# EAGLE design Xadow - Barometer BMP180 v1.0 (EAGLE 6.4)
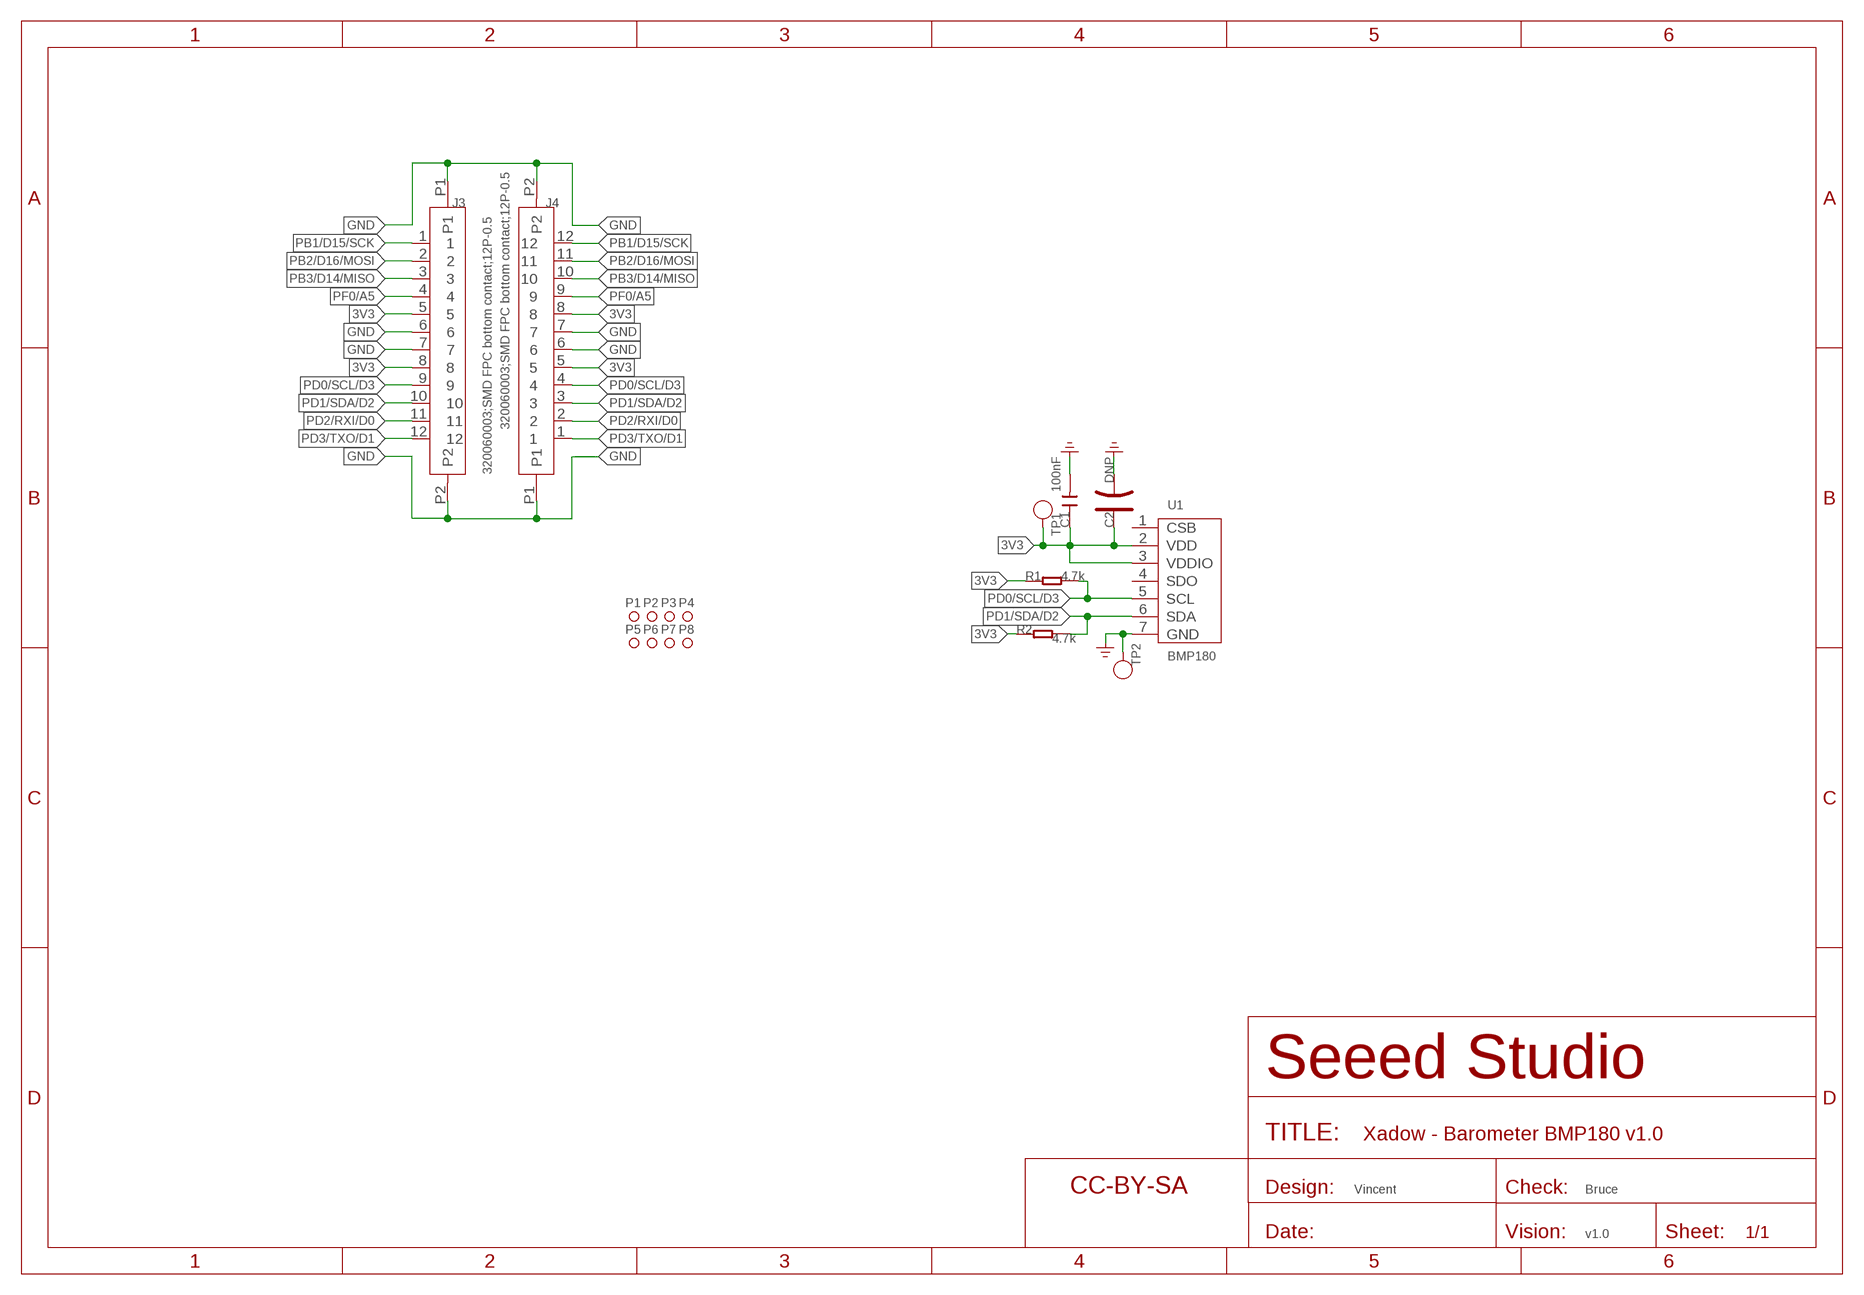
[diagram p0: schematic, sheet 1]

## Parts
C1  100nF  CAP-0603  [C0603]
C2  DNP  CAP-POLAR-AVX-A  [AVX-A]
J3  320060003;SMD FPC bottom contact;12P-0.5  FPC-CONNECTOR-12P-FH12-12S-0.5SH  [12P-0.5]
J4  320060003;SMD FPC bottom contact;12P-0.5  FPC-CONNECTOR-12P-FH12-12S-0.5SH  [12P-0.5]
P1  PAD-MARK'ANNULAR'  [ROUND-MARK-1.0]
P2  PAD-MARK'ANNULAR'  [ROUND-MARK-1.0]
P3  PAD-MARK'ANNULAR'  [ROUND-MARK-1.0]
P4  PAD-MARK'ANNULAR'  [ROUND-MARK-1.0]
P5  PAD-MARK'ANNULAR'  [ROUND-MARK-1.0]
P6  PAD-MARK'ANNULAR'  [ROUND-MARK-1.0]
P7  PAD-MARK'ANNULAR'  [ROUND-MARK-1.0]
P8  PAD-MARK'ANNULAR'  [ROUND-MARK-1.0]
R1  4.7k  RES-0603  [R0603]
R2  4.7k  RES-0603  [R0603]
TP1  PAD-TEST-POINT'4545'  [TP-D45MIL]
TP2  PAD-TEST-POINT'4545'  [TP-D45MIL]
U1  BMP180  [LGA-7]
U$1  SEEEDSTUDIO-OPEN-SCH-FRAME  [SEEEDSTUDIO-PCB-FRAME]

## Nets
3V3: C1.1 C2.+ J3.5 J3.8 J4.5 J4.8 R1.1 R2.1 TP1.T U1.2(VDD) U1.3(VDDIO)
GND: C1.2 C2.- J3.6 J3.7 J3.P1 J3.P2 J4.6 J4.7 J4.P1 J4.P2 TP2.T U1.7(GND) ; supply symbol labelled GND_POWER
PB1/D15/SCK: J3.1 J4.12
PB2/D16/MOSI: J3.2 J4.11
PB3/D14/MISO: J3.3 J4.10
PD0/SCL/D3: J3.9 J4.4 R1.2 U1.5(SCL)
PD1/SDA/D2: J3.10 J4.3 R2.2 U1.6(SDA)
PD2/RXI/D0: J3.11 J4.2
PD3/TXO/D1: J3.12 J4.1
PF0/A5: J3.4 J4.9
Unconnected: U1.1(CSB) U1.4(SDO)

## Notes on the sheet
- Vincent | Bruce
- v1.0

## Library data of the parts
C1 = Discrete-new:CAP: Ceramic Capacitors
C2 = Discrete-new:CAP-POLAR: Electrolytic Capacitors,Tantalum Capacitors and Super Capacitors
J3 J4 = Connector-new:FPC-CONNECTOR-12P: 320060003
P1-P8 = Discrete-new:PAD-MARK; PARTNO: DNP
R1 R2 = Discrete-new:RES
TP1 TP2 = Discrete-new:PAD-TEST-POINT; PARTNO: DNP
U1 = template:BMP180: Digital pressure sensor
U$1 = moudle-new:SEEEDSTUDIO-OPEN-SCH-FRAME

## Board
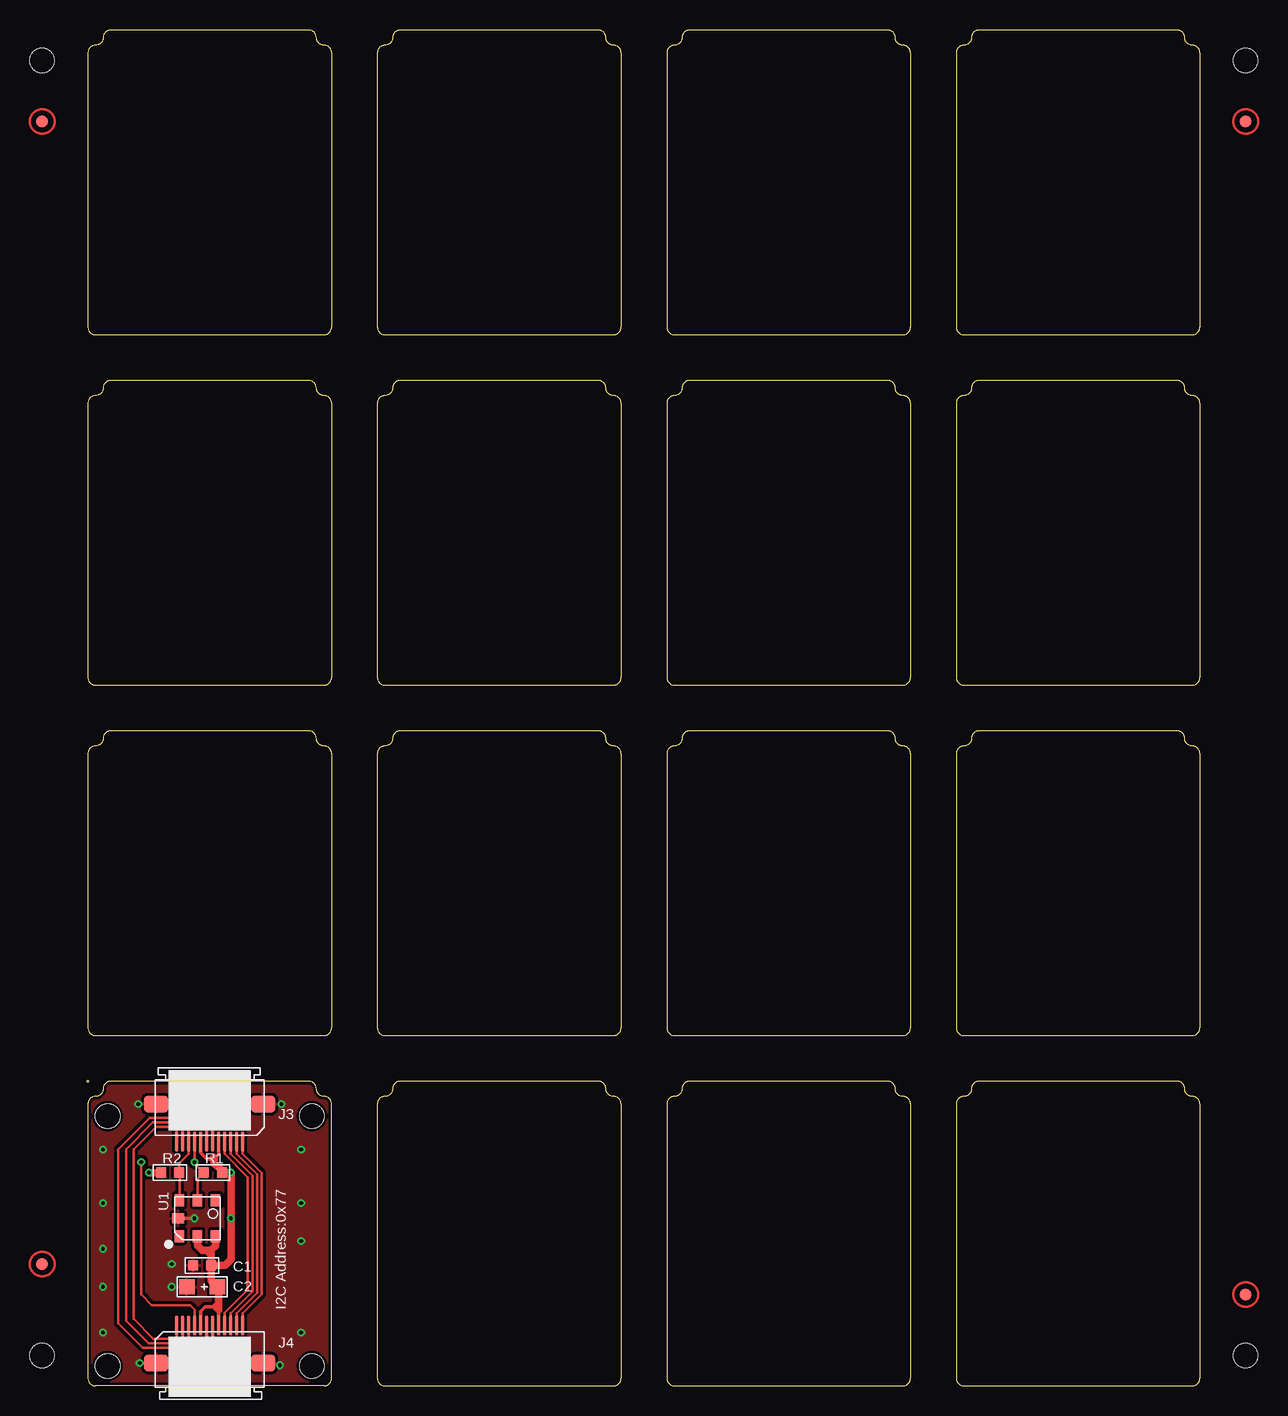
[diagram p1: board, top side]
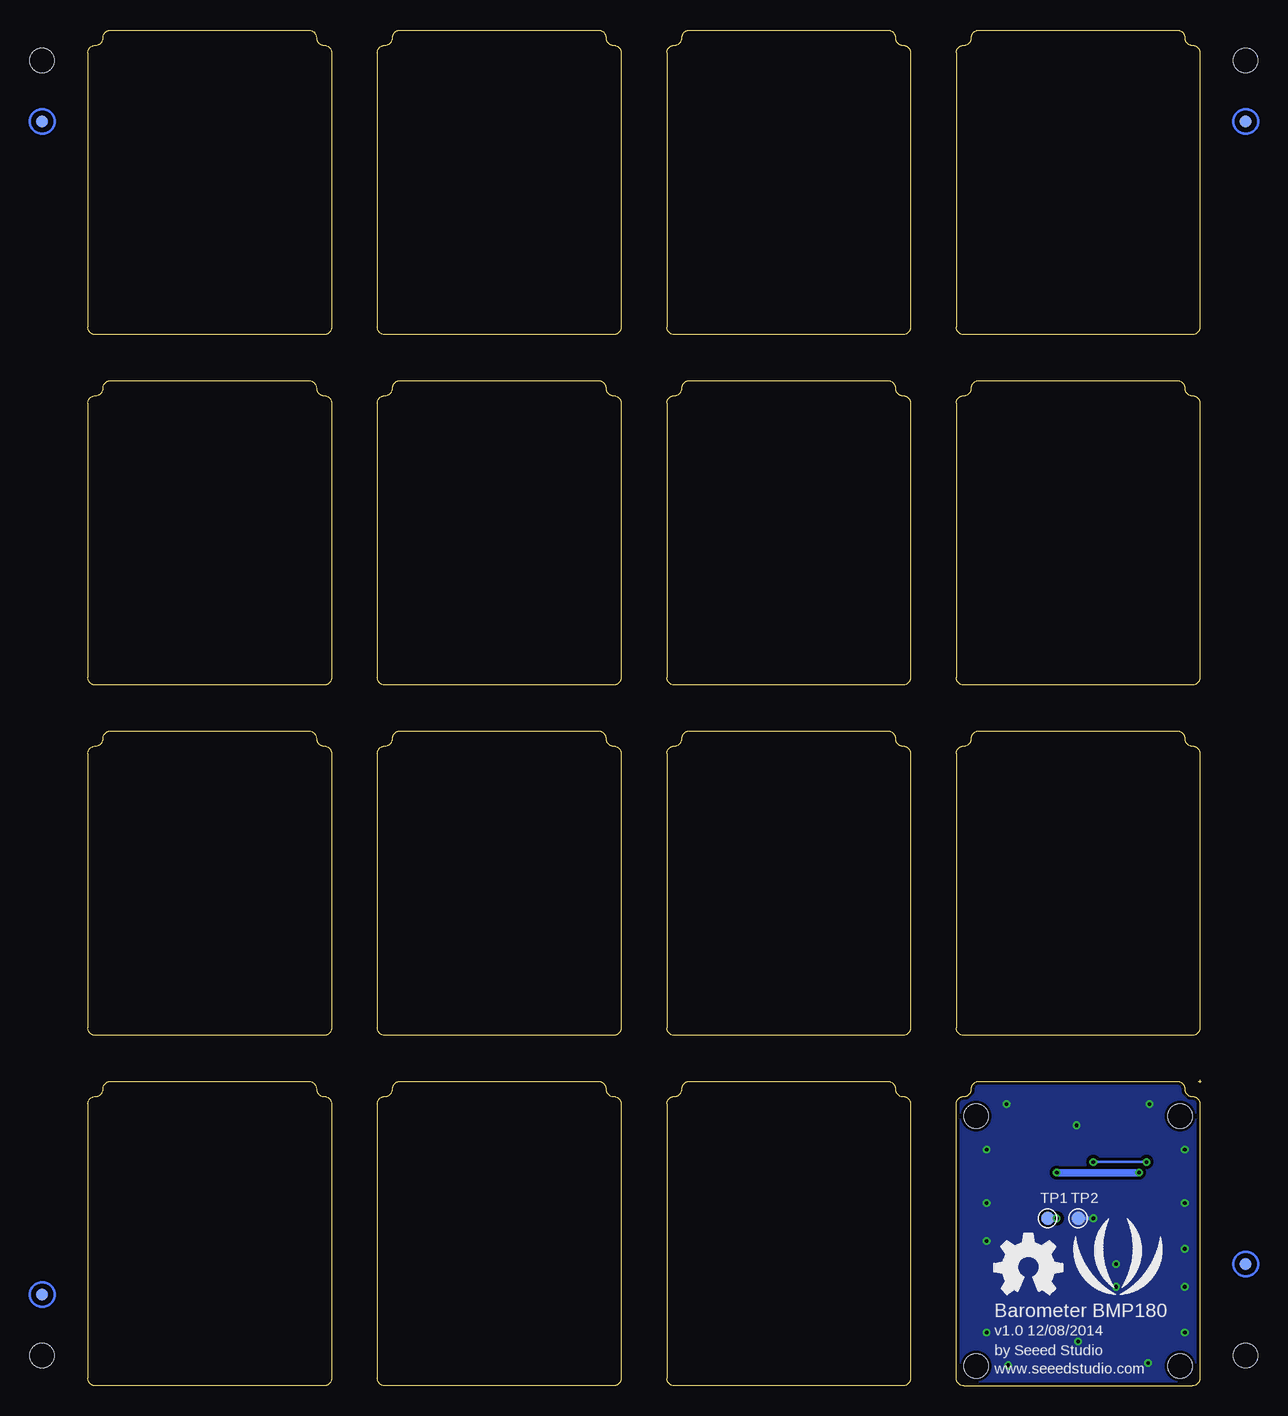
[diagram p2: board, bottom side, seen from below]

Size 92.84 x 113.03 mm. Coordinates in mm from the lower left corner, seen from the top.
Outline: 180 segments
Copper layers (1*16): Top 0.035mm / dielectric 1.5mm / Bottom 0.035mm
Design rules "SeeedStudio_2layer_DRU_no_angle_20140221 *": minimum track width 6mil, minimum drill 12mil, track to track 6mil, track to pad 6mil, pad to pad 6mil, via to via 6mil, smd to smd 0mil, copper to edge 10mil, drill to drill 10mil, minimum pad ring 10mil, minimum via ring 6mil, stop-mask expansion 2mil, vias tented up to drill 25mil, thermal gap 10mil
Holes 2.03 mm at -3.68,110.49 -3.68,2.54 96.65,2.54 96.65,110.49

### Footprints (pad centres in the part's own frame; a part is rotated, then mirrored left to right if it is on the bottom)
C0603 = smd 0.889 x 0.889: 1 0,0.762; 2 0,-0.762
AVX-A = smd 1.27 x 1.27: + -1.27,0; - 1.27,0
12P-0.5 = smd 0.3 x 1.6: 1 -2.75,3.127; 2 -2.25,3.127; 3 -1.75,3.127; 4 -1.25,3.127; 5 -0.75,3.127; 6 -0.25,3.127; 7 0.25,3.127; 8 0.75,3.127; 9 1.25,3.127; 10 1.75,3.127; 11 2.25,3.127; 12 2.75,3.127 | smd 2.032 x 1.397: P1 -4.445,0; P2 4.445,0
ROUND-MARK-1.0 = smd 1.016 x 1.016: P$1 0,0
R0603 = smd 0.889 x 0.889: 1 0,0.762; 2 0,-0.762
TP-D45MIL = smd 1.143 x 1.143: T 0,0
LGA-7 = smd 0.8 x 1: 1 1.5,1.5; 2 0,1.5; 3 -1.5,1.5; 4 -1.5,-1.5; 5 0,-1.5; 6 1.5,-1.5 | smd 1 x 0.8: 7 1.6,0
XADOW-DRILL-DIM-25*20MM = hole 2.032: -9.779,-8.509; -9.779,8.509; 11.049,8.509; 11.049,-8.509

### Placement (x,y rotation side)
C1  9.65,10.03 270 top
C2  9.65,8.26 180 top
J3  10.29,23.5 180 top
J4  10.29,1.91 0 top
P1  not placed on the board
P2  not placed on the board
P3  not placed on the board
P4  not placed on the board
P5  not placed on the board
P6  not placed on the board
P7  not placed on the board
P8  not placed on the board
R1  10.54,17.78 270 top
R2  6.99,17.78 90 top
TP1  12.83,13.97 0 bottom
TP2  10.29,13.97 0 bottom
U1  9.27,13.97 180 top
U$1  not placed on the board
U$5  [OSHW_FILLX200_NOTEXT]  17.27,7.62 0 bottom
U$6  [SEEED_LOGO250]  10.67,7.62 0 bottom
U$7  [XADOW-DRILL-DIM-25*20MM]  10.29,12.7 270 top

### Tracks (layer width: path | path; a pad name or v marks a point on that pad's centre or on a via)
3V3  (via drill 0.3 pad 0.64)
  Top 0.305: J4.8 11.04,6.34 11.05,6.35 | J3.5 11.04,19.29 10.67,18.92 10.29,18.92 | J3.8 9.54,19.42 10.03,18.92 10.29,18.92 | J4.5 9.54,6.24 9.91,6.6 10.54,6.6 | 10.54,6.6 11.05,6.6 11.18,6.73 11.05,6.73 | 10.54,6.6 10.92,6.99 | 10.54,6.6 10.92,6.22 | 10.29,18.92 10.54,19.18 | 10.29,18.92 10.54,18.67
  Top 0.61: C1.1 10.41,8.76 C2.+ 11.05,8.13 11.05,6.73 11.05,6.35 | U1.3 10.77,11.68 10.41,11.33 10.41,11.3 | C1.1 10.41,11.3 | U1.2 9.27,11.68 9.65,11.3 10.03,11.3 | 10.03,11.3 10.41,11.3 | 10.03,11.3 10.29,11.05 | C1.1 11.56,10.03 12.07,10.54 v12.07,13.97 v12.07,17.78 R1.1 11.3,17.91 10.67,18.54 10.67,18.92 10.67,19.05 | R2.1 v5.21,17.78
  Bottom 0.61: v5.21,17.78 v12.07,17.78 | v12.07,13.97 TP1.T
GND  (via drill 0.3 pad 0.64)
  Top 0.305: J4.7 10.54,3.93 v10.29,3.68 10.04,3.93 J4.6 | J3.6 10.54,21.59 v10.41,21.72 10.04,21.34 J3.7 | U1.7 v9.02,13.97
  Bottom 0.305: TP2.T v9.02,13.97
  other vias: 16.26,23.5 7.11,8.26 7.11,10.16 16.13,1.71 4.45,1.91 4.32,23.5 1.4,4.45 1.4,8.26 1.4,11.43 1.4,15.24 1.4,19.68 17.91,4.45 17.91,15.24 17.91,19.68 17.91,12.06
  pour Top (isolate 0.254, rank 6): -0.51,26.04 21.08,26.04 21.08,-0.64 -0.51,-0.64
  pour Bottom (isolate 0.254, rank 6): -0.51,26.04 21.08,26.04 21.08,-0.64 -0.51,-0.64
PB1/D15/SCK
  Top 0.203: J4.12 13.04,6.05 14.61,7.62 14.61,17.78 13.04,19.35 J3.1
PB2/D16/MOSI
  Top 0.203: J4.11 12.54,6.06 14.22,7.75 14.22,17.65 12.54,19.34 J3.2
PB3/D14/MISO
  Top 0.203: J4.10 12.04,6.07 13.84,7.87 13.84,17.53 12.04,19.33 J3.3
PD0/SCL/D3  (via drill 0.3 pad 0.64)
  Top 0.203: U1.5 9.27,17.27 R1.2 9.04,18.52 9.04,18.69 | J4.4 9.04,6.33 8.64,6.73 5.46,6.73 4.57,7.62 v4.57,18.67 | J3.9 9.04,18.69 | 9.04,18.69 v9.02,18.67
  Bottom 0.203: v4.57,18.67 v9.02,18.67
PD1/SDA/D2
  Top 0.203: U1.6 7.77,17.76 R2.2 7.75,18.54 8.54,19.33 J3.10 8.54,21.56 7.75,22.35 5.29,22.35 2.67,19.73 2.67,5.22 4.72,3.17 8,3.17 8.54,3.71 J4.3
PD2/RXI/D0
  Top 0.203: J4.2 8.04,3.97 7.62,3.56 5.18,3.56 3.3,5.43 3.3,19.72 5.55,21.97 7.49,21.97 8.04,21.43 J3.11
PD3/TXO/D1
  Top 0.203: J3.12 7.54,21.29 7.24,21.59 5.83,21.59 3.94,19.7 3.94,5.59 5.59,3.94 7.37,3.94 7.54,4.11 J4.1
PF0/A5
  Top 0.203: J4.9 11.54,6.08 13.46,8 13.46,17.4 11.54,19.32 J3.4

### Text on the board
tPlace: I2C Address:0x77
bPlace: Barometer BMP180 | v1.0 12/08/2014 | by Seeed Studio | www.seeedstudio.com

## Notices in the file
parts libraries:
moudle-new: This work is licensed under the Creative Commons Attribution 4.0 International License.
To view a copy of this license,visit:
http://creativecommons.org/licenses/by-sa/4.0
moudle-new: CC-BY-SA
